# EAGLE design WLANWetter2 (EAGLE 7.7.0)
ABBREV: rf1; PROJECT: RFM12B Board
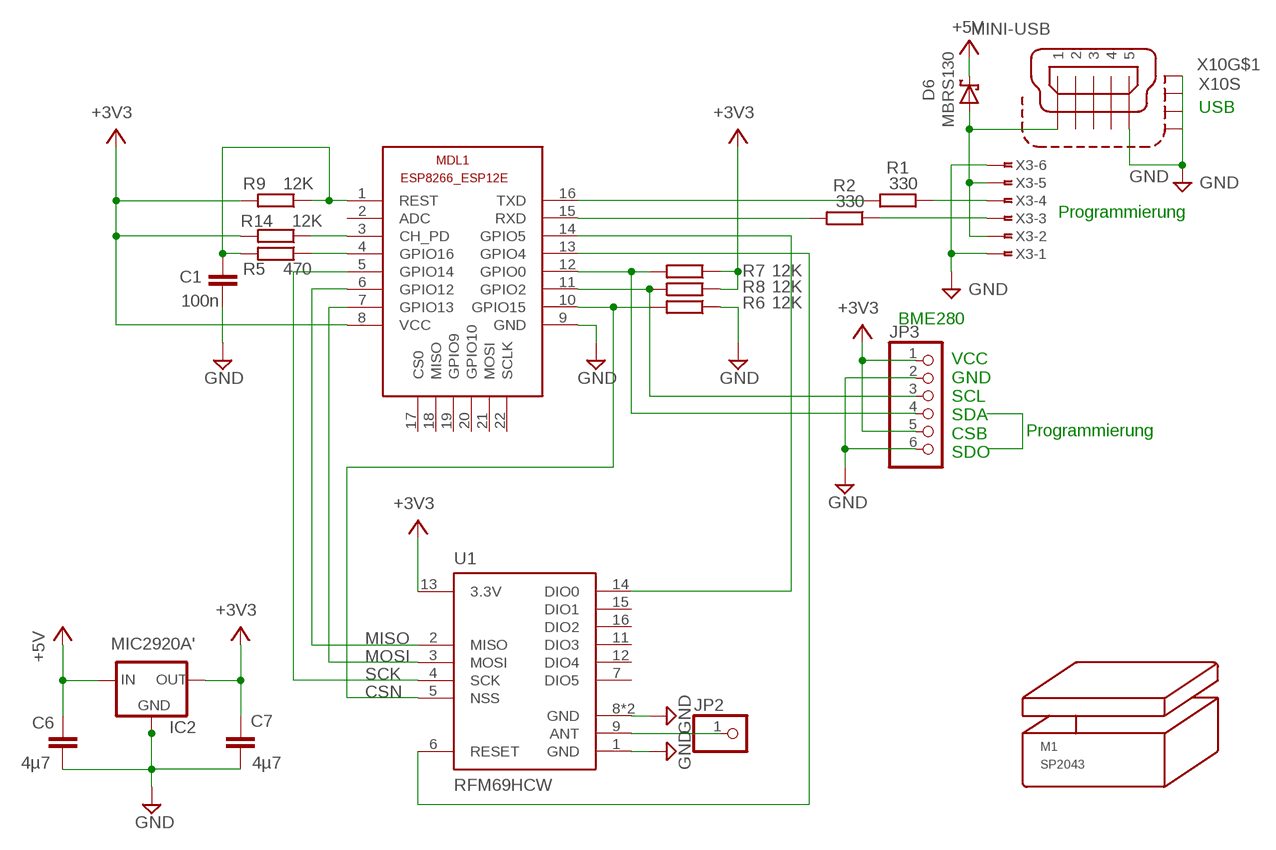
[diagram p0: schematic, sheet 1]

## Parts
C1  100n  C-EUC0805  [C0805]
C6  4µ7  C-EUC0805  [C0805]
C7  4µ7  C-EUC0805  [C0805]
D6  MBRS130  MBRS130LT3  [SMB]
IC2  MIC2920A'  [SOT223]
JP2  PINHD-1X1  [1X01]
JP3  PINHD-1X6  [1X06]
M1  SP2043  [SP2043]
MDL1  ESP8266-12EESP8266-ESP12E  [ESP8266-ESP12E]
R1  330  R-EU_R0805  [R0805]
R2  330  R-EU_R0805  [R0805]
R5  470  R-EU_R0805  [R0805]
R6  12K  R-EU_R0805  [R0805]
R7  12K  R-EU_R0805  [R0805]
R8  12K  R-EU_R0805  [R0805]
R9  12K  R-EU_R0805  [R0805]
R14  12K  R-EU_R0805  [R0805]
U1  RFM69HCW  [RFM69HCW-XXXS2]
X3  FTOP-6+H  [FTOP-6-A]
X10  MINI-USB  MINI-USB-SCHIELD-32005-201  [32005-201]

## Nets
+3V3: C7.2 IC2.3(OUT) JP3.1 JP3.5 MDL1.8(VCC) R7.1 R8.1 R9.2 R14.2 U1.13(3.3V)
+5: D6.2(A1) X3.2 X3.5 X10.1
+5V: C6.2 D6.1(K1) IC2.1(IN)
ANT: JP2.1 U1.9(ANT)
CSN: MDL1.10(GPIO15) R6.2 U1.5(NSS)
GND [power]: C1.1 C6.1 C7.1 IC2.2(GND) IC2.4(GND) JP3.2 JP3.6 MDL1.9(GND) R6.1 U1.1(GND) U1.8(GND) U1.10(GND) X3.1 X3.6 X10.5 X10.M1(S:S1) X10.M2(S:S2) X10.M3(S:S3) X10.M4(S:S4)
MISO: MDL1.6(GPIO12) U1.2(MISO)
MOSI: MDL1.7(GPIO13) U1.3(MOSI)
N$2: MDL1.13(GPIO4) U1.6(RESET)
N$3: MDL1.14(GPIO5) U1.14(DIO0)
N$8: MDL1.4(GPIO16) R5.1
N$12: C1.2 MDL1.1(REST) R5.2 R9.1
N$14: MDL1.3(CH_PD) R14.1
N$29: R1.1 X3.4
N$30: R2.1 X3.3
RX: MDL1.15(RXD) R2.2
SCK: MDL1.5(GPIO14) U1.4(SCK)
SCL: JP3.3 MDL1.11(GPIO2) R8.2
SDA: JP3.4 MDL1.12(GPIO0) R7.2
TX: MDL1.16(TXD) R1.2
Unconnected: MDL1.2(ADC) MDL1.17(CS0) MDL1.18(MISO) MDL1.19(GPIO9) MDL1.20(GPIO10) MDL1.21(MOSI) MDL1.22(SCLK) U1.7(DIO5) U1.11(DIO3) U1.12(DIO4) U1.15(DIO1) U1.16(DIO2) X10.2 X10.3 X10.4

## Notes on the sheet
- USB
- Programmierung
- BME280
- Programmierung
- VCC
  GND
  SCL
  SDA
  CSB
  SDO

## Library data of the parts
C1 C6 C7 = rcl:C-EU: CAPACITOR, European symbol
D6 = m-glmini:MBRS130LT3
IC2 = m-glmini:MIC2920A'
JP2 = pinhead:PINHD-1X1: PIN HEADER
JP3 = pinhead:PINHD-1X6: PIN HEADER
M1 = strapubox:SP2043: Gehäuse Strapubox Typ 2043
MDL1 = ESP8266-ESP12E:ESP8266-12E: ESP8266-12E with additional I/O and GPIO04/05 corrected The author cannot warrant that this library is free from error or will meet your specific requirements. Created by PuceBaboon.com. Komagane, Nagano, JAPAN
R1 R2 R5-R9 R14 = rcl:R-EU_: RESISTOR, European symbol
U1 = mike-temp:RFM69H
X3 = con-amp_a:FTOP-6: AMP Federleiste 215079
X10 = con-cypressindustries:MINI-USB-SCHIELD-: MINI USB-B Conector Source: www.cypressindustries.com

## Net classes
1 power: width 0.203 mm, drill 0.305 mm, clearance 0.152 mm

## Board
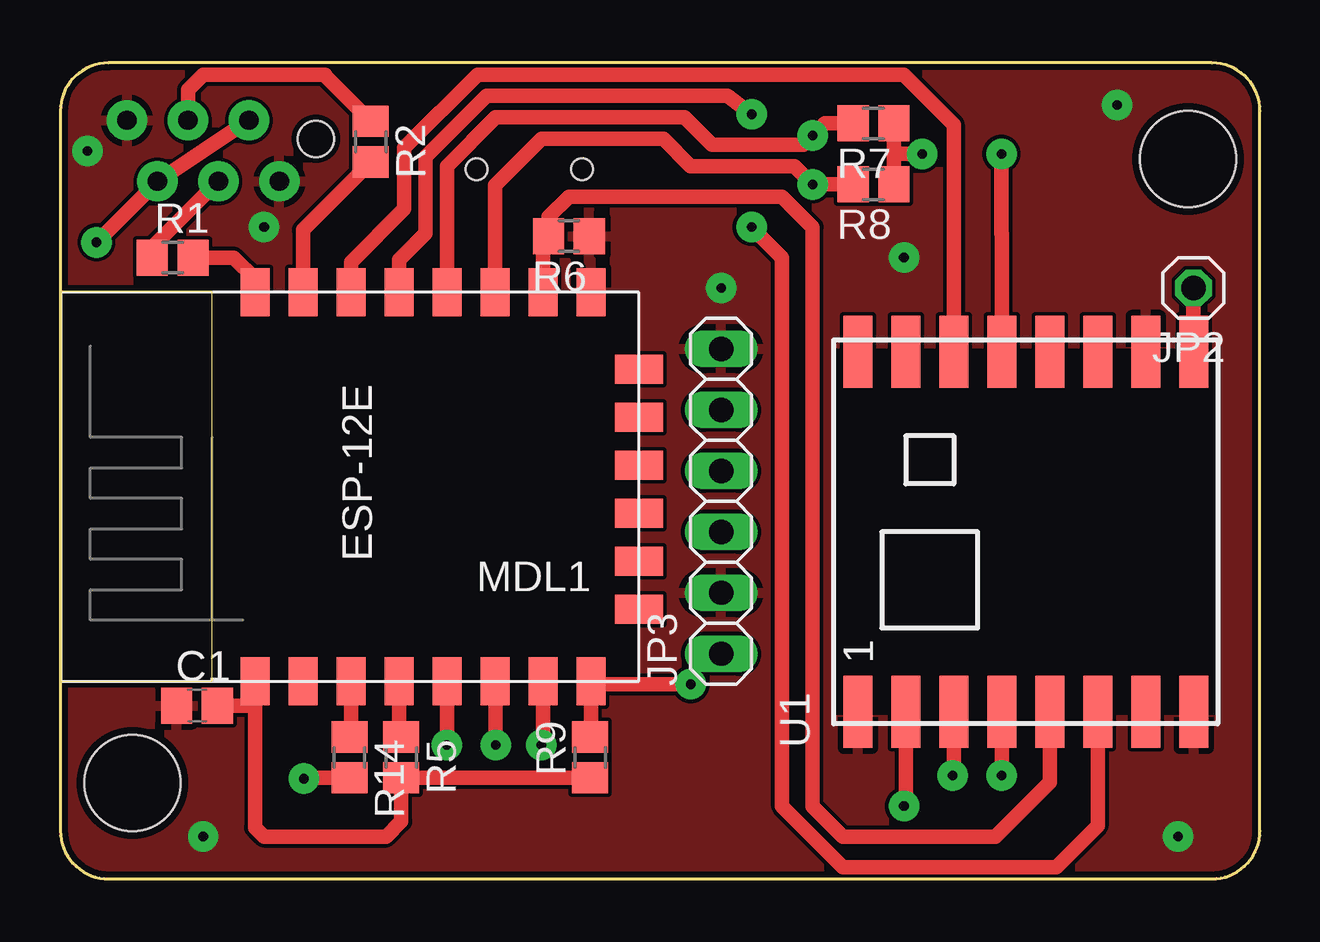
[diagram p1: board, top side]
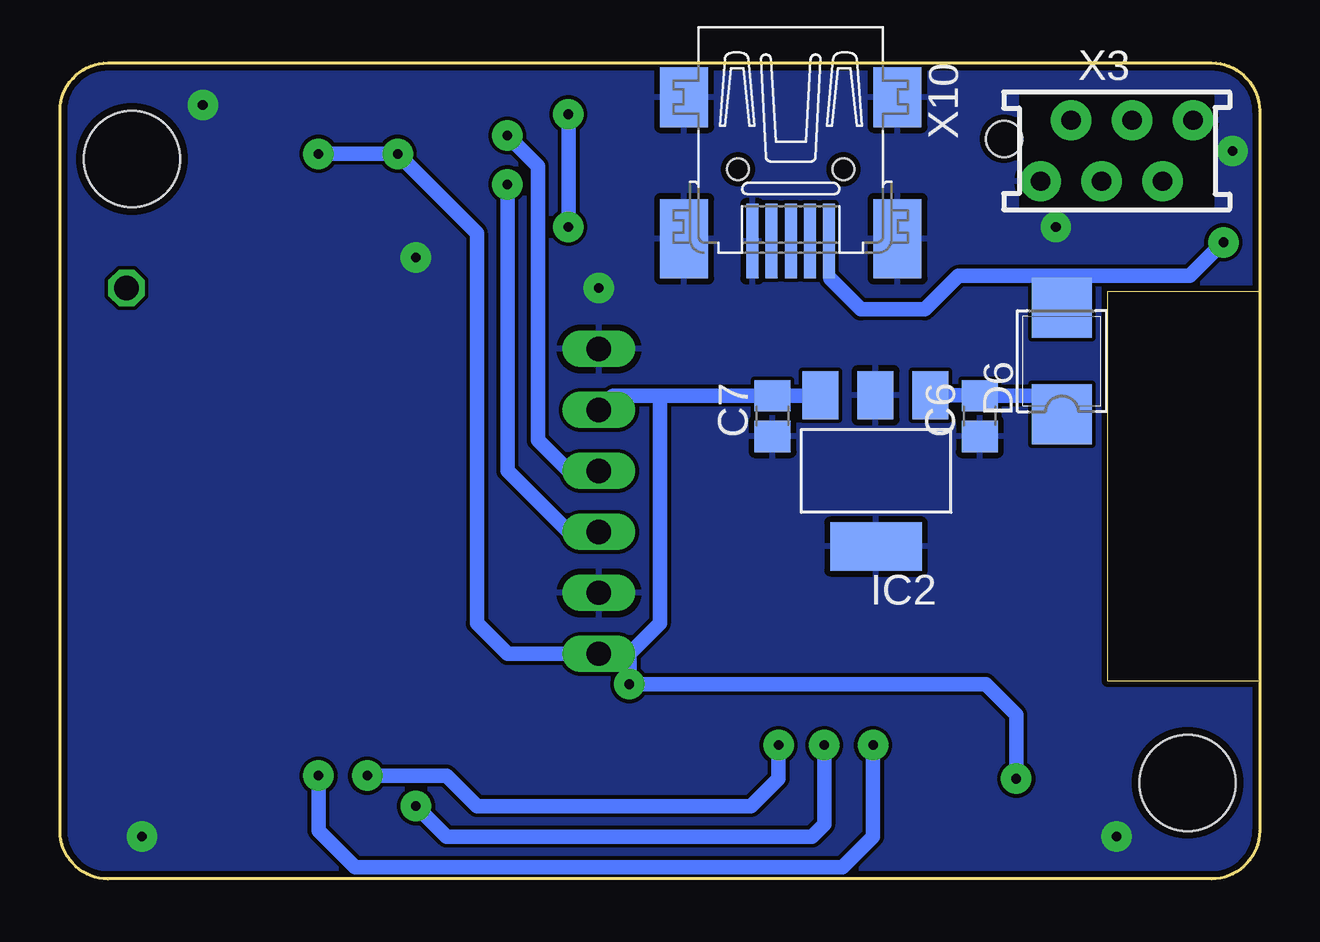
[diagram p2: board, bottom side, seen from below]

Size 50.02 x 34 mm. Coordinates in mm from the lower left corner, seen from the top.
Outline: 0,8.24 6.35,8.24 6.35,24.49 0,24.49
Copper layers (1*16): Top 0.035mm / dielectric 1.5mm / Bottom 0.035mm
Design rules "SeeedStudio_2layer_DRU_no_angle_20140221 *": minimum track width 6mil, minimum drill 12mil, track to track 6mil, track to pad 10mil, pad to pad 10mil, via to via 6mil, smd to smd 0mil, copper to edge 10mil, drill to drill 10mil, minimum pad ring 10mil, minimum via ring 6mil, stop-mask expansion 2mil, vias tented up to drill 100mil, thermal gap 10mil
tRestrict: area 0,8.2 to 24.1,24.5; area 32.3,6.8 to 48.3,22.1
bRestrict: area -0.4,8.1 to 6.3,24.6; area 1.9,27.8 to 10,32.9

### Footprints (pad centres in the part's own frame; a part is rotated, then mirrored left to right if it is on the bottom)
C0805 = smd 1.3 x 1.5: 1 -0.85,0; 2 0.85,0
SMB = smd 2.5 x 2.5: 1 -2.22,-0.001; 2 2.223,0.001
SOT223 = smd 1.499 x 2.007: 1 -2.261,-3.15; 2 0.025,-3.15; 3 2.311,-3.15 | smd 3.81 x 2.007: 4 0,3.15
1X01 = drill 1.016 octagon: 1 0,0
1X06 = drill 1.016 long: 1 -6.35,0; 2 -3.81,0; 3 -1.27,0; 4 1.27,0; 5 3.81,0; 6 6.35,0
SP2043 = hole 4: -22,-13; 22,13
ESP8266-ESP12E = smd 2 x 1.2: 1 0,16; 2 0,14; 3 0,12; 4 0,10; 5 0,8; 6 0,6; 7 0,4; 8 0,2; 9 16.2,2; 10 16.2,4; 11 16.2,6; 12 16.2,8; 13 16.2,10; 14 16.2,12; 15 16.2,14; 16 16.2,16 | smd 1.2 x 2: 17 11,0; 18 3,0; 19 5,0; 20 13,0; 21 7,0; 22 9,0
R0805 = smd 1.3 x 1.5: 1 -0.85,0; 2 0.85,0
RFM69HCW-XXXS2 = smd 3 x 1.2: 1 -7.5,7; 2 -7.5,5; 3 -7.5,3; 4 -7.5,1; 5 -7.5,-1; 6 -7.5,-3; 7 -7.5,-5; 8 -7.5,-7; 9 7.5,-7; 10 7.5,-5; 11 7.5,-3; 12 7.5,-1; 13 7.5,1; 14 7.5,3; 15 7.5,5; 16 7.5,7
FTOP-6-A = drill 0.8 pad 1.676: 1 3.175,1.27; 2 1.905,-1.27; 3 0.635,1.27; 4 -0.635,-1.27; 5 -1.905,1.27; 6 -3.175,-1.27 | hole 1.5: -4.7,0.5
32005-201 = smd 3.1 x 0.5: 1 3,1.6; 2 3,0.8; 3 3,0; 4 3,-0.8; 5 3,-1.6 | smd 2.5 x 2: M1 -3,-4.45; M2 -3,4.45 | smd 3.3 x 2: M3 2.9,4.45; M4 2.9,-4.45 | hole 0.9: 0,2.2; 0,-2.2

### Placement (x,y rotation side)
C1  5.71,7.22 0 top
C6  11.68,19.29 90 bottom
C7  20.32,19.29 90 bottom
D6  8.25,21.57 90 bottom
IC2  16,17 180 bottom
JP2  47.24,24.62 180 top
JP3  27.56,15.73 90 top
M1  25.02,17 180 top
MDL1  24.13,8.24 90 top
R1  4.7,25.89 0 top
R2  12.95,30.72 270 top
R5  14.22,5.06 270 top
R6  21.21,26.78 180 top
R7  33.91,31.48 180 top
R8  33.91,28.94 180 top
R9  22.1,5.06 90 top
R14  12.06,5.06 270 top
U1  40.26,14.46 90 top
X3  5.97,30.33 0 bottom
X10  19.56,29.57 270 bottom

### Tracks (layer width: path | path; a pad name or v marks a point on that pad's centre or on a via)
+3V3  (via drill 0.4 pad 1.27)
  Top 0.61: R9.2 22.13,5.91 MDL1.8 22.26,8.11 v26.29,8.11 | R14.2 10.16,4.21 v10.16,4.17 | U1.13 39.26,26.89 39.24,26.89 v39.24,30.21 | R8.1 R7.1 34.76,30.21 v35.94,30.21
  Bottom 0.61: v10.16,4.17 10.16,6.84 11.43,8.11 v26.29,8.11 26.29,9.38 | IC2.3 18.33,20.14 C7.2 25.02,20.14 | 25.02,20.14 26.96,20.14 JP3.5 | 25.02,20.14 25.02,10.65 26.29,9.38 | 26.29,9.38 JP3.1 31.37,9.38 32.64,10.65 32.64,26.91 v35.94,30.21 v39.24,30.21
+5  (via drill 0.4 pad 1.27)
  Top 0.61: X3.5 X3.2 v1.52,26.52
  Bottom 0.406: 17.91,25 17.91,26.52 X10.1
  Bottom 0.61: v1.52,26.52 2.92,25.13 8.26,25.13 | 8.26,25.13 12.57,25.13 13.97,23.73 16.64,23.73 17.91,25 | D6.2 8.26,25.13
+5V
  Bottom 0.61: D6.1 9.04,20.14 C6.2 11.7,20.15 IC2.1
ANT
  Top 0.61: U1.9 47.24,21.96 JP2.1
CSN
  Top 0.61: U1.5 41.26,4.03 38.99,1.76 32.64,1.76 31.37,3.03 31.37,27.16 30.1,28.43 21.21,28.43 20.36,27.58 R6.2 20.13,26.55 MDL1.10
GND  (via drill 0.4 pad 1.27)
  other vias: 1.14,30.33 8.51,27.16 44.07,32.24 46.61,1.76 5.97,1.76 35.18,25.89 27.56,24.62
  pour Bottom: 50.55,-0.78 -0.25,-0.78 -0.25,34.78 50.55,34.78
  pour Bottom: 12.19,10.65 12.19,14.46 19.81,14.46 19.81,10.65
  pour Top: 51.82,-2.05 -1.52,-2.05 -1.52,36.05 51.82,36.05
MISO  (via drill 0.4 pad 1.27)
  Top 0.61: MDL1.6 18.16,8.21 v18.16,5.57 | v35.18,3.03 35.26,3.11 U1.2
  Bottom 0.61: v18.16,5.57 18.16,2.27 18.67,1.76 33.91,1.76 v35.18,3.03
MOSI  (via drill 0.4 pad 1.27)
  Top 0.61: MDL1.7 20.13,5.63 v20.07,5.57 | v37.21,4.3 37.26,4.35 U1.3
  Bottom 0.61: v20.07,5.57 20.07,4.17 21.21,3.03 32.64,3.03 33.91,4.3 v37.21,4.3
N$2  (via drill 0.4 pad 1.27)
  Top 0.61: U1.6 43.26,2.22 41.53,0.49 32.64,0.49 30.1,3.03 30.1,25.89 v28.83,27.16 | MDL1.13 14.13,25.8 15.24,26.91 15.24,30.08 17.78,32.62 27.81,32.62 v28.83,31.86
  Bottom 0.61: v28.83,31.86 v28.83,27.16
N$3
  Top 0.61: MDL1.14 12.13,25.7 14.35,27.92 14.35,30.46 17.4,33.51 35.18,33.51 37.26,31.43 U1.14
N$8
  Top 0.61: R5.1 14.13,5.91 MDL1.4
N$12
  Top 0.61: MDL1.1 8.13,7.22 | 8.13,7.22 8.13,2.14 8.51,1.76 13.59,1.76 14.22,2.39 R5.2 R9.1 | C1.2 8.13,7.22
N$14
  Top 0.61: R14.1 12.13,5.91 MDL1.3
N$29
  Top 0.61: R1.1 3.85,26.31 X3.4
N$30
  Top 0.61: X3.3 5.33,32.88 5.97,33.51 11.05,33.51 11.05,33.47 R2.1
RX
  Top 0.61: R2.2 10.13,27.04 MDL1.15
SCK  (via drill 0.4 pad 1.27)
  Top 0.61: MDL1.5 v16.13,5.57 | v39.24,4.3 39.26,4.32 U1.4
  Bottom 0.61: v16.13,5.57 16.13,1.76 17.4,0.49 37.72,0.49 39.24,2.01 v39.24,4.3
SCL  (via drill 0.4 pad 1.27)
  Top 0.61: MDL1.11 18.13,28.91 20.07,30.84 25.15,30.84 26.29,29.7 30.61,29.7 v31.37,28.94 R8.2 32.13,28.94
  Bottom 0.61: JP3.3 28.83,14.46 31.37,17 v31.37,28.94
SDA  (via drill 0.4 pad 1.27)
  Top 0.61: MDL1.12 16.13,29.7 18.16,31.73 26.04,31.73 27.18,30.59 30.99,30.59 v31.37,30.97 31.88,31.48 R7.2
  Bottom 0.61: JP3.4 28.83,17 30.1,18.27 30.1,29.7 v31.37,30.97
TX
  Top 0.61: MDL1.16 8.13,25 7.24,25.89 R1.2

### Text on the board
_tNames: J3 | J2 | R2 | R4 | C4 | R3 | R1 | C5 | C2 | MAX31865 | FB1 | LED | C3 | FB2
_bNames: PT100 | P2W | P3 | P2/3W
_bFinish: P3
